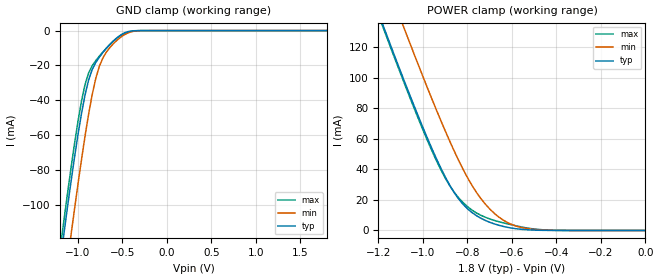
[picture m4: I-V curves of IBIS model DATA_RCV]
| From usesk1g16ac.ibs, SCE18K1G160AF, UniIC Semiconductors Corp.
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|   Model DATA_RCV
[Model]  DATA_RCV
Model_type Input
Polarity   Non-Inverting
Vinl = 360.000mV
Vinh = 1440.000mV
C_comp   2.0990pF   2.0750pF   2.3110pF
[Temperature Range]   25.0000   70.0000   0.0
[Voltage Range]   1.8000V   1.7000V   1.9000V
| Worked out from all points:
|   GND clamp passes 1 mA (typ) near -0.46 V on its own axis
|   POWER clamp passes 1 mA (typ) near -0.57 V on its own axis
[GND_clamp]
|Voltage   I(typ)   I(min)   I(max)
-1.8V     -382.1mA   -414.5mA   -375.5mA
-1.2V     -133.2mA   -165.3mA   -125.6mA
-1.16V    -117.7mA   -149.4mA   -110mA
-1.08V    -87.61mA   -118.3mA   -79.77mA
-1V       -59.95mA   -88.41mA   -52.3mA
-920mV    -36.92mA   -60.6mA    -30.96mA
-880mV    -28.39mA   -48.02mA   -24.34mA
-800mV    -18.4mA    -27.56mA   -17.29mA
-680mV    -10.16mA   -12.34mA   -10.08mA
-520mV    -2.567mA   -3.816mA   -2.802mA
-280mV    -6.329uA   -40.92uA   -18.02uA
1.8V      3.312nA    86.13nA    3.394nA
[POWER_clamp]
|Voltage   I(typ)   I(min)   I(max)
-1.8V     384.7mA    419.1mA    384.4mA
-1.18V    134.5mA    169.2mA    133.2mA
-1.16V    126.8mA    161.4mA    125.5mA
-1.08V    96.37mA    130.6mA    94.93mA
-960mV    53.65mA    86.15mA    52.25mA
-880mV    29.71mA    58.57mA    29.39mA
-840mV    20.7mA     45.97mA    21.4mA
-780mV    11.76mA    29.58mA    13.37mA
-680mV    4.343mA    11.31mA    6.611mA
-600mV    1.533mA    3.842mA    3.663mA
-520mV    368.6uA    1.001mA    1.353mA
0V        3.312nA    53.68nA    3.878nA
